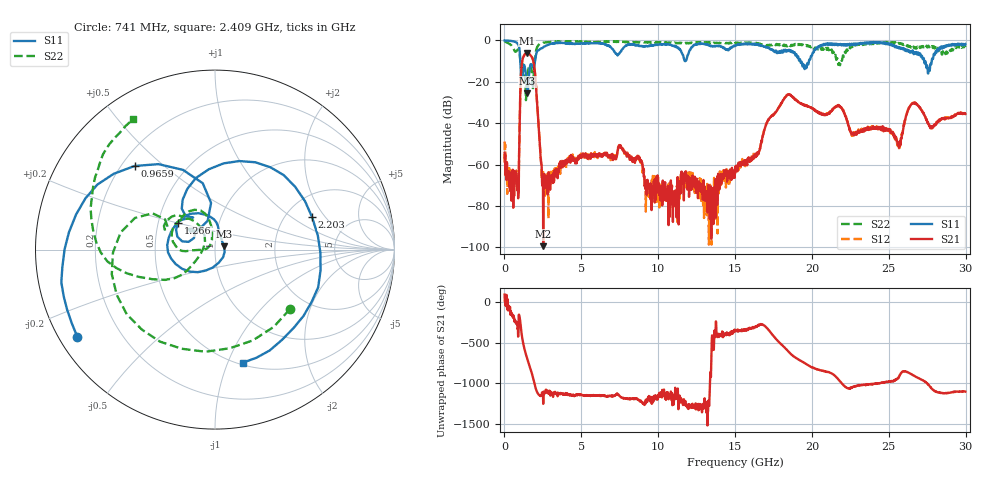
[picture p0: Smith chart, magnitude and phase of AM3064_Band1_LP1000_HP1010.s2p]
# Hz S DB R 50.0
!freq dBS11 angS11 dBS21 angS21 dBS12 angS12 dBS22 angS22
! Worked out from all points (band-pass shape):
!   1600 points, 10 MHz to 29.98 GHz, reference 50 ohm
!   highest |S21| = -6.01 dB at 1.472 GHz (marker M1); lowest = -99.5 dB at 2.522 GHz (marker M2)
!   |S21| within 3 dB of the highest: 1.183 GHz to 1.839 GHz (656.3 MHz wide, 43.4 % of centre)
!   lowest |S11| = -25.5 dB at 1.491 GHz (marker M3), VSWR 1.11, Z = 55.2 + j1.95 ohm
!   |S11| at or under -10 dB: 1.031 GHz to 1.989 GHz (958.4 MHz wide, 63.5 % of centre); 19.25 GHz to 19.8 GHz (555.8 MHz wide, 2.85 % of centre); 27.3 GHz to 27.79 GHz (488.5 MHz wide, 1.77 % of centre)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
!   |S22| runs from -28.9 to -0.4 dB; largest |S21 - S12| = 0.0058
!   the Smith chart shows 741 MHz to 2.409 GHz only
!   S11 on the Smith chart (normalised r, x): 741 MHz: 0.05, -0.29; 965.9 MHz: 0.25, +0.40; 1.266 GHz: 0.63, +0.20; 2.203 GHz: 2.78, +1.48; 2.409 GHz: 0.52, -1.13
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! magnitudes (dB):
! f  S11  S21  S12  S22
! 10 MHz  0.0  -54.3  -48.8  -0.4
! 741 MHz  -0.8  -63.2  -65.6  -5.5
! 965.9 MHz  -3.8  -49.8  -49.1  -5.4
! 1.266 GHz  -11.9  -7.4  -7.4  -12.1
! 1.472 GHz  -24.4  -6.0  -6.0  -18.8
! 1.491 GHz  -25.5  -6.0  -6.0  -17.1
! 1.884 GHz  -13.3  -10.2  -10.2  -18.3
! 2.203 GHz  -4.9  -39.4  -39.2  -2.3
! 2.409 GHz  -3.8  -59.7  -65.4  -1.3
! 2.522 GHz  -3.3  -99.5  -64.4  -1.1
! 5.015 GHz  -1.4  -56.7  -55.9  -0.8
! 7.582 GHz  -5.4  -51.7  -52.0  -0.7
! 10 GHz  -2.0  -70.1  -66.3  -0.9
! 13.52 GHz  -2.9  -73.7  -78.6  -1.3
! 15 GHz  -2.7  -63.9  -64.1  -1.5
! 18.34 GHz  -5.4  -26.7  -26.7  -2.5
! 19.99 GHz  -7.4  -32.8  -32.8  -3.1
! 25 GHz  -1.4  -43.4  -43.3  -1.1
! 25.67 GHz  -3.8  -51.8  -52.1  -1.4
! 26.63 GHz  -6.6  -30.4  -30.3  -3.1
! 27.56 GHz  -16.0  -40.1  -40.4  -2.7
! 29.98 GHz  -1.7  -35.5  -35.5  -3.2
